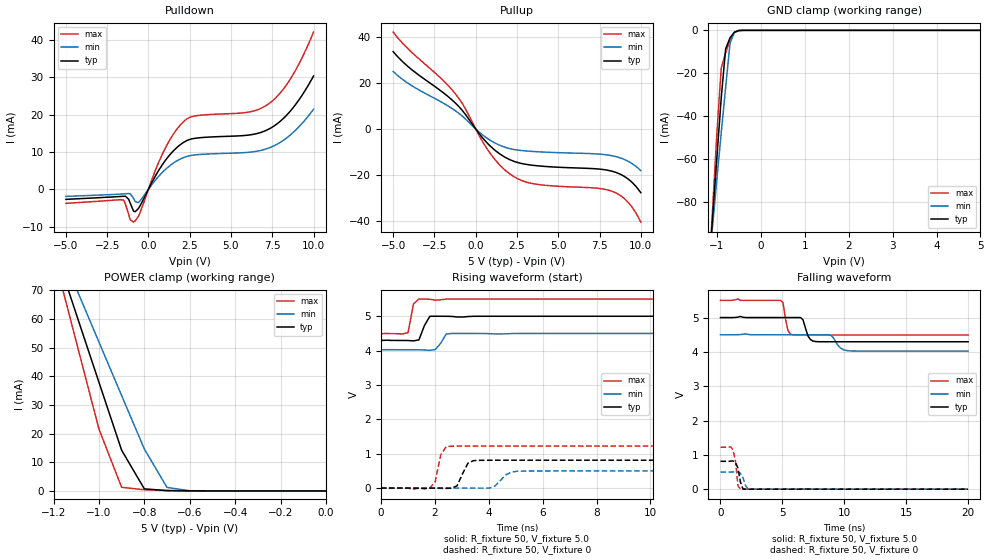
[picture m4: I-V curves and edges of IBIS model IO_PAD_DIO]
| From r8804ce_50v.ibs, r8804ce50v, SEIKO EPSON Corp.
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[Model]   IO_PAD_DIO
Model_type I/O
Enable Active-High
Polarity Non-Inverting
Vinh=4.4
Vinl=0.9
Vmeas=2.50
C_comp   2.5p   2.0p   3.0p
[Temperature Range] 25   105   -40
[Voltage Range]   5.0   4.5   5.5
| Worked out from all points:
|   slope of the pulldown table from 0 to 0.75 V, typ, clamps not added: 126 ohm
|   slope of the pullup table from 0 to 0.75 V, typ, clamps not added: 116 ohm
|   GND clamp passes 1 mA (typ) near -0.61 V on its own axis
|   POWER clamp passes 1 mA (typ) near -0.80 V on its own axis
|   falling waveform, R_fixture 50, V_fixture 5.0: 20-80 % time 392ps typ, 551ps min, 301ps max; typ from 5 V to 4.29 V
|   falling waveform, R_fixture 50, V_fixture 0: 20-80 % time 288ps typ, 327ps min, 256ps max; typ from 0.812 V to 0 V
|   rising waveform, R_fixture 50, V_fixture 5.0: 20-80 % time 240ps typ, 249ps min, 146ps max; typ from 4.29 V to 5 V
|   rising waveform, R_fixture 50, V_fixture 0: 20-80 % time 300ps typ, 387ps min, 200ps max; typ from 0 V to 0.812 V
[Pullup]
-5V       33.52mA    24.92mA    42mA
-3.9V     25.87mA    18.88mA    33.39mA
-2.1V     16.45mA    11.75mA    21.92mA
-1.2V     11.01mA    7.73mA     14.97mA
-800mV    7.926mA    5.5mA      10.92mA
800mV     -6.847mA   -4.548mA   -9.793mA
2V        -13.08mA   -8.393mA   -19.13mA
2.7V      -14.84mA   -9.282mA   -22.1mA
3.5V      -15.78mA   -9.765mA   -23.74mA
8.3V      -18.4mA    -11.66mA   -27.12mA
9.2V      -21.51mA   -13.88mA   -31.53mA
10V       -27.61mA   -18.03mA   -40.4mA
[Pulldown]
-5V       -2.695mA   -1.898mA   -3.76mA
-1.5V     -1.871mA   -1.232mA   -2.909mA
-1.1V     -3.756mA   -1.223mA   -8.145mA
-900mV    -5.868mA   -2.416mA   -8.805mA
-600mV    -5.116mA   -3.564mA   -7.202mA
900mV     6.952mA    4.772mA    9.936mA
2V        12.16mA    8.239mA    17.55mA
2.7V      13.56mA    9.131mA    19.52mA
6.1V      14.53mA    9.907mA    20.68mA
7.3V      16.12mA    11.06mA    22.91mA
8.6V      20.95mA    14.55mA    29.52mA
10V       30.3mA     21.42mA    42.06mA
[GND Clamp]
-5V       -1.258A    -1.018A    -1.574A
-1.2V     -117.3mA   -114.6mA   -121.6mA
-1.1V     -88.33mA   -91.95mA   -84.56mA
-1V       -59.57mA   -69.57mA   -48.26mA
-900mV    -31.49mA   -47.77mA   -17.61mA
-800mV    -8.683mA   -26.7mA    -10.45mA
-700mV    -3.453mA   -6.033mA   -4.512mA
-600mV    -868.8uA   -930.5uA   -956.3uA
-500mV    -86.23uA   -135.6uA   -52.66uA
-400mV    -4.725uA   -14.69uA   -1.074uA
5V        49.11pA    6.071uA    26.26pA
[POWER Clamp]
-5V       999.8mA    810.1mA    1.25A
-1.2V     85.6mA     89.47mA    82.67mA
-1.1V     61.75mA    70.7mA     52.12mA
-1V       37.96mA    51.97mA    21.63mA
-900mV    14.22mA    33.28mA    1.266mA
-800mV    725.6uA    14.64mA    407.5uA
-700mV    111.9uA    1.216mA    132.2uA
-600mV    21.56uA    73.28uA    21.07uA
0V        49.11pA    1.092nA    32.97pA
[Falling Waveform]
R_fixture=50
V_fixture=5.0
V_fixture_min=4.5
V_fixture_max=5.5
0s        5V         4.5V       5.5V
4.848ns   5V         4.5V       5.5V
5.051ns   5V         4.5V       5.437V
5.455ns   5V         4.5V       4.617V
5.859ns   5V         4.5V       4.496V
6.667ns   4.937V     4.5V       4.492V
7.071ns   4.463V     4.5V       4.492V
7.677ns   4.301V     4.5V       4.492V
10.3ns    4.295V     4.034V     4.492V
20ns      4.295V     4.024V     4.492V
[Falling Waveform]
R_fixture=50
V_fixture=0
V_fixture_min=0
V_fixture_max=0
0s        811.5mV    498.6mV    1.223V
808.1ps   816.3mV    497.6mV    1.235V
1.01ns    822.5mV    501.8mV    1.154V
1.212ns   779.8mV    507.4mV    822.7mV
1.414ns   615.3mV    501.7mV    99.47mV
1.616ns   206.5mV    458.1mV    811uV
1.818ns   4.626mV    333.6mV    92.59uV
2.02ns    333.4uV    109.8mV    13.18uV
2.222ns   52.34uV    4.521mV    9.345uV
20ns      0V         0V         1.155uV
[Rising Waveform]
R_fixture=50
V_fixture=5.0
V_fixture_min=4.5
V_fixture_max=5.5
0s        4.295V     4.024V     4.492V
1.01ns    4.294V     4.024V     4.521V
1.212ns   4.283V     4.024V     5.359V
1.414ns   4.312V     4.024V     5.5V
1.616ns   4.726V     4.019V     5.5V
1.818ns   5V         4.008V     5.495V
2.02ns    5V         4.032V     5.468V
2.424ns   4.999V     4.482V     5.498V
2.626ns   4.995V     4.5V       5.5V
20ns      5V         4.5V       5.5V
[Rising Waveform]
R_fixture=50
V_fixture=0
V_fixture_min=0
V_fixture_max=0
0s        0V         0V         0V
1.818ns   -665.5uV   218.6uV    -2.885mV
2.02ns    70.19uV    -1.935mV   194mV
2.222ns   86.63uV    -8.277mV   964.9mV
2.626ns   -2.751mV   -14.96uV   1.219V
3.434ns   798.2mV    -65.72uV   1.223V
4.04ns    810.5mV    1.402mV    1.223V
4.646ns   811.4mV    389.2mV    1.223V
5.253ns   811.5mV    494.7mV    1.223V
20ns      811.5mV    498.6mV    1.223V
[Ramp]
R_load=50
dV/dt_r   4.869E-1/2.539E-10   2.992E-1/3.669E-10   7.336E-1/1.940E-10
dV/dt_f   4.228E-1/3.598E-10   2.856E-1/5.439E-10   6.049E-1/2.505E-10
|[End   IO_PAD_DIO
